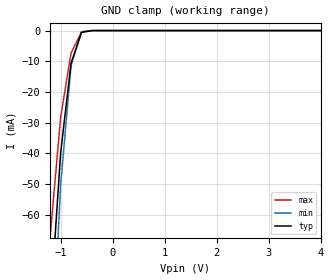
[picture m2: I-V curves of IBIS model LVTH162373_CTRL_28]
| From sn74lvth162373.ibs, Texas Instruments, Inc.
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|   Model LVTH162373 Input_CTRL_28
[Model]   LVTH162373_CTRL_28
Model_type  Input
Polarity   Inverting
Vinl = 0.8V
Vinh = 2.0V
| variable   typ   min   max
C_comp   3p   NA   NA
[Temperature Range]   25   -40   85
[Voltage range]   2.8   2.7   2.9
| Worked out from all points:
|   GND clamp passes 1 mA (typ) near -0.61 V on its own axis
|Process range|   weak   strong
[GND Clamp]
|   25C:2.8V   -40C:2.7V   85C:2.9V
|   Voltage   I(typ)   I(min)   I(max)
-5V       -1.632A    -1.922A    -1.465A
-1.2V     -90.82mA   -118.2mA   -66.69mA
-1V       -39.73mA   -50.13mA   -28.17mA
-800mV    -10.61mA   -11.44mA   -7.314mA
-600mV    -601.7uA   -368.3uA   -461uA
-400mV    -1.299uA   -933nA     -1.654uA
5V        -163.1pA   182.4nA    297.4pA
